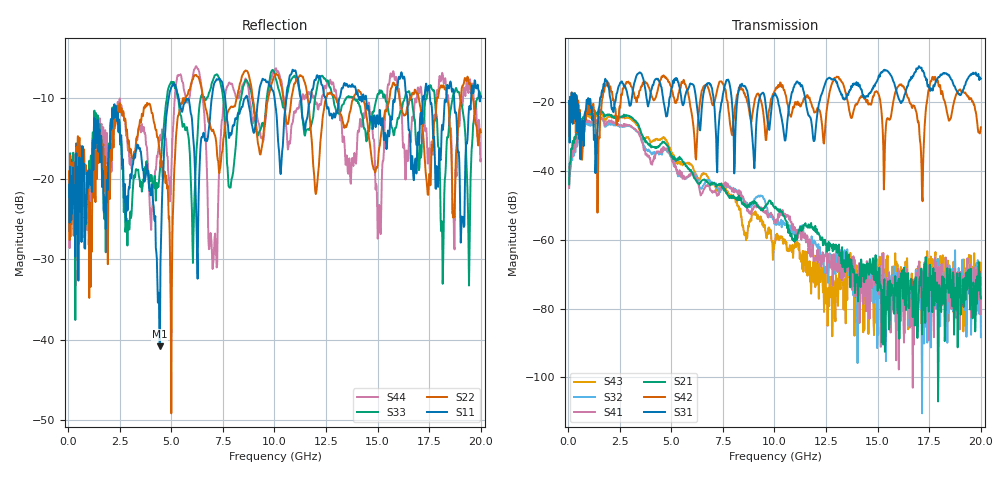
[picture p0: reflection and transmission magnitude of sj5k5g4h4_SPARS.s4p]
! FILE: E:\users\goganessyan\GBX_Backplane\FR408_backplane\1m_INBOUND_FEXT\sj5k5g4h4_SPARS.s4p
# MHZ S RI R 50.00
! FREQ  S11  S12  S13  S14
!  S21  S22  S23  S24
!  S31  S32  S33  S34
!  S41  S42  S43  S44
!  REAL  IMAG  REAL  IMAG  REAL  IMAG  REAL  IMAG
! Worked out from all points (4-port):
!   799 points, 50 MHz to 20 GHz, reference 50 ohm
!   strongest paths, dB at 50 MHz, 5.025 GHz, 10.03 GHz, 15.03 GHz, 20 GHz:
!     S31: -19.7, -15.6, -17.4, -13.1, -13.2
!     S42: -19.8, -16.5, -16.6, -17.5, -27.3
!     S21: -43.9, -35.9, -50.9, -70.9, -77.1
!     S41: -44.9, -36.8, -54.3, -73.4, -81.7
!     S32: -44.9, -35.9, -54.8, -87.6, -88.3
!     S43: -43.0, -34.9, -60.9, -73.3, -73.0
!   lowest |S11| = -40.8 dB at 4.45 GHz (marker M1), VSWR 1.02, Z = 50.9 + j0.08 ohm
!   |S11| at or under -10 dB: start of sweep to 4.873 GHz; 5.361 GHz to 6.96 GHz (1.599 GHz wide, 26 % of centre); 14.44 GHz to 15.84 GHz (1.394 GHz wide, 9.21 % of centre)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
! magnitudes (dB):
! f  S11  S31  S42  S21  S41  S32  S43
! 50 MHz  -20.7  -19.7  -19.8  -43.9  -44.9  -44.9  -43.0
! 4.45 GHz  -40.8  -14.4  -13.8  -32.4  -34.5  -34.8  -31.0
! 5.075 GHz  -8.3  -14.5  -17.5  -36.2  -37.1  -36.6  -35.5
! 9 GHz  -14.3  -36.8  -21.0  -49.6  -50.4  -48.8  -52.7
! 12.65 GHz  -11.8  -12.9  -17.7  -63.1  -66.5  -66.1  -79.3
! 18.12 GHz  -13.3  -11.9  -16.8  -70.7  -79.0  -77.8  -66.6
! 20 GHz  -9.7  -13.2  -27.3  -77.1  -81.7  -88.3  -73.0
